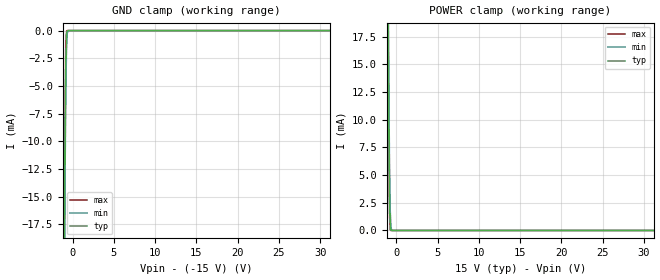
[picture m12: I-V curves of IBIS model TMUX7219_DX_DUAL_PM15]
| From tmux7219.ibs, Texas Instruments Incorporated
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[Model]   TMUX7219_DX_DUAL_PM15
Model_type   Terminator
|   typ   min   max
C_comp   49pF   49pF   49pF
[Voltage Range]   30   27   33
[Temperature Range]   27   125   -40
[Power Clamp Reference]   15   15   15
[GND Clamp Reference]   -15   -15   -15
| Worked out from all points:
|   GND clamp passes 1 mA (typ) near -0.77 V on its own axis
|   POWER clamp passes 1 mA (typ) near -0.77 V on its own axis
[GND Clamp]
|   Voltage   I(typ)   I(min)   I(max)
-30V      -4.646A    -4.64A     -4.649A
-1.02V    -22.01mA   -24.41mA   -19.81mA
-930mV    -11.04mA   -13.89mA   -8.565mA
-840mV    -3.269mA   -5.934mA   -1.414mA
-750mV    -384.6uA   -1.761mA   -36.1uA
-660mV    -13.98uA   -270.8uA   -470.3nA
-570mV    -401.3nA   -19.98uA   -235.2nA
-210mV    0A         0A         0A
60V       0A         0A         0A
[POWER Clamp]
|   Voltage   I(typ)   I(min)   I(max)
-30V      4.646A     4.64A      4.649A
-1.02V    22.01mA    24.41mA    19.81mA
-930mV    11.04mA    13.89mA    8.565mA
-840mV    3.269mA    5.934mA    1.414mA
-750mV    384.6uA    1.761mA    36.1uA
-660mV    13.98uA    270.8uA    470.3nA
-570mV    401.3nA    19.98uA    235.2nA
-210mV    0A         0A         0A
60V       0A         0A         0A
